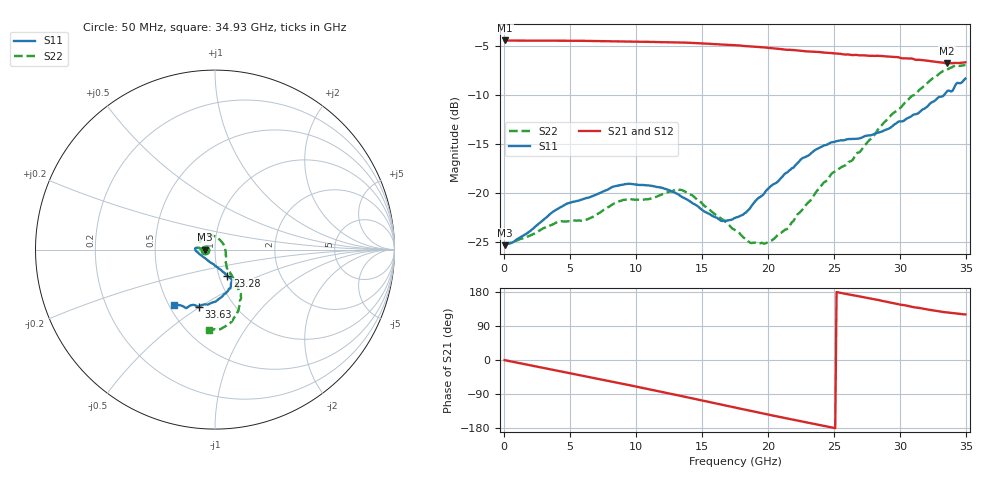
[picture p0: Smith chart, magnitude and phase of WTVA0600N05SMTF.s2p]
! 50 ohm 2-Port S-parameters measured by Modelithics Inc support@modelithics.com  Tampa, FL USA 813-866-6335 (February 2024)
! Smiths Interconnect,  6dB P/N: WTVA0600N05SMTF, Temperature: 75 C
! Board: 10 mil Rogers 4350B, Mounting Pad Dimensions: Length: 15 mils, Width: 25 mils, Gap: 40 mils.
# Hz S RI R 50
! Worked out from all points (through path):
!   352 points, 50 MHz to 34.93 GHz, reference 50 ohm
!   highest |S21| = -4.45 dB at 100 MHz (marker M1); lowest = -6.8 dB at 33.53 GHz (marker M2)
!   group delay of S21, straight-line fit = 19.7 ps
!   lowest |S11| = -25.3 dB at 50 MHz (marker M3), VSWR 1.11, Z = 44.9 + j0.0339 ohm
!   |S11| at or under -10 dB: start of sweep to 33.32 GHz
!   |S22| runs from -25.4 to -7.0 dB; largest |S21 - S12| = 0.0064
!   S11 on the Smith chart (normalised r, x): 50 MHz: 0.90, +0.00; 23.28 GHz: 1.10, -0.33; 33.63 GHz: 0.69, -0.49; 34.93 GHz: 0.53, -0.38
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5e7  -0.0541 0.000376  0.5988 -0.00337  0.5981 -0.00327  -0.0535 -0.00132
1e8  -0.0545 -6.64e-05  0.5988 -0.00739  0.5984 -0.00741  -0.0547 -0.000945
2.986e9  -0.0725 0.00548  0.5598 -0.2098  0.559 -0.2104  -0.066 -0.00391
4.6775e9  -0.0874 0.00749  0.5042 -0.32  0.5036 -0.3196  -0.0713 -0.00521
5.8715e9  -0.0919 0.00976  0.4515 -0.3897  0.451 -0.3895  -0.0722 -0.00199
9.155e9  -0.1105 0.00772  0.2595 -0.5322  0.2589 -0.5316  -0.0906 0.0168
1.1742e10  -0.1067 -0.00684  0.0758 -0.5823  0.0744 -0.5818  -0.0806 0.0539
1.36325e10  -0.0924 -0.019  -0.0666 -0.5802  -0.0676 -0.5794  -0.0626 0.0809
1.64185e10  -0.0519 -0.0502  -0.2621 -0.5075  -0.2627 -0.5066  -0.000643 0.0742
1.7513e10  -0.0317 -0.0675  -0.3289 -0.4616  -0.3292 -0.4605  0.0195 0.0613
1.8707e10  -0.00425 -0.0851  -0.3901 -0.3987  -0.3903 -0.3975  0.0415 0.0368
1.98015e10  0.0164 -0.1004  -0.4372 -0.3354  -0.4369 -0.3346  0.0547 0.00856
2.1493e10  0.0417 -0.121  -0.4845 -0.2303  -0.4843 -0.2289  0.0595 -0.0286
2.3284e10  0.0682 -0.1447  -0.5128 -0.1157  -0.5121 -0.116  0.0596 -0.0715
2.33835e10  0.0702 -0.1463  -0.5141 -0.1095  -0.5134 -0.1093  0.0603 -0.0739
2.4876e10  0.0859 -0.1598  -0.5156 -0.0132  -0.515 -0.0121  0.0686 -0.1065
2.6667e10  0.0954 -0.1628  -0.497 0.0936  -0.496 0.0948  0.0855 -0.1337
2.91545e10  0.0884 -0.1937  -0.4391 0.2304  -0.4361 0.2342  0.128 -0.206
3.1841e10  0.0327 -0.2669  -0.3337 0.3365  -0.3314 0.3375  0.1329 -0.3265
3.35325e10  -0.0867 -0.3177  -0.2668 0.3722  -0.2634 0.3738  0.0663 -0.4199
3.3632e10  -0.0915 -0.3198  -0.2641 0.3747  -0.2605 0.3766  0.0616 -0.4248
3.49255e10  -0.2275 -0.308  -0.2331 0.4007  -0.2322 0.4001  -0.0354 -0.4472
